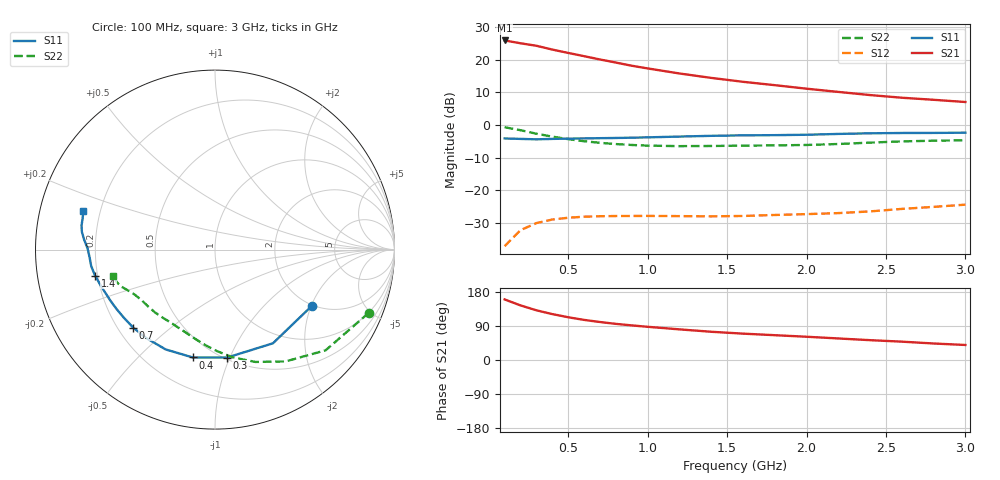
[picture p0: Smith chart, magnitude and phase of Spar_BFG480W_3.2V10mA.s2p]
! Filename: 3_210BFG480.001
! Title: BFG480W
! Bias: Vce=3.2V; Ic=10mA
! Company: NXP Semiconductors NL
! User: Quality&Reliability T&D
! Measure time: 10 Nov 1999 / 11:56:12
#  MHz  S  MA  R 50
! Freq  S11  S21  S12  S22  :
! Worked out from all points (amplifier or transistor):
!   20 points, 100 MHz to 3 GHz, reference 50 ohm
!   highest |S21| = 25.8 dB at 100 MHz (marker M1)
!   |S21| within 3 dB of that: start of sweep to 421.2 MHz
!   unconditionally stable (mu >= 1): 1.692 GHz to end of sweep
!   at 400 MHz: K = 0.23, MSG = 26.0 dB, |S12| = -28.9 dB
!   at 1.2 GHz: K = 0.73, MSG = 21.8 dB, |S12| = -27.8 dB
!   at 3 GHz: K = 1.17, MAG = 13.2 dB, |S12| = -24.3 dB
!   S11 on the Smith chart (normalised r, x): 100 MHz: 1.96, -2.02; 300 MHz: 0.52, -0.98; 400 MHz: 0.38, -0.74; 700 MHz: 0.26, -0.38; 1.4 GHz: 0.19, -0.10; 3 GHz: 0.14, +0.14
100  0.6239 -30.2  19.58 159.8  0.01411 69.9  0.926 -22.4
200  0.6138 -58.3  17.74 144.1  0.02477 57.1  0.8335 -42.3
300  0.6051 -83.5  16.25 131.1  0.03175 47.6  0.7369 -57.7
400  0.6135 -101.6  14.22 121.1  0.03604 40.5  0.6652 -70.2
500  0.6205 -116.3  12.63 112.8  0.03832 35.7  0.6083 -80.7
600  0.6243 -127.9  11.27 105.8  0.03977 32.6  0.5657 -88.9
700  0.6299 -136.4  10.03 100.3  0.04043 30.5  0.535 -95.8
800  0.6341 -143.4  9.004 95.3  0.04073 29.4  0.5119 -101.7
900  0.6406 -148.8  8.051 91.3  0.04081 29.2  0.4958 -107.0
1000  0.6483 -153.9  7.325 87.6  0.04092 29.2  0.4847 -112.0
1200  0.6663 -162.0  6.131 80.8  0.04061 30.5  0.4758 -120.9
1400  0.6838 -167.8  5.251 74.5  0.04028 33.0  0.4785 -128.1
1600  0.6958 -172.4  4.575 69.6  0.04081 37.1  0.4841 -133.8
1800  0.7005 -176.7  4.065 65.5  0.04227 41.9  0.4888 -139.3
2000  0.7104 179.4  3.591 61.4  0.04356 46.8  0.496 -145.1
2200  0.7312 175.7  3.205 56.9  0.04514 50.8  0.513 -150.8
2400  0.7478 172.5  2.87 52.3  0.04793 54.5  0.5386 -155.3
2600  0.7556 169.8  2.612 48.4  0.05233 57.7  0.5624 -158.6
2800  0.7574 167.0  2.429 43.5  0.05619 59.5  0.576 -161.6
3000  0.7637 163.7  2.247 39.6  0.06077 61.4  0.5853 -165.4
